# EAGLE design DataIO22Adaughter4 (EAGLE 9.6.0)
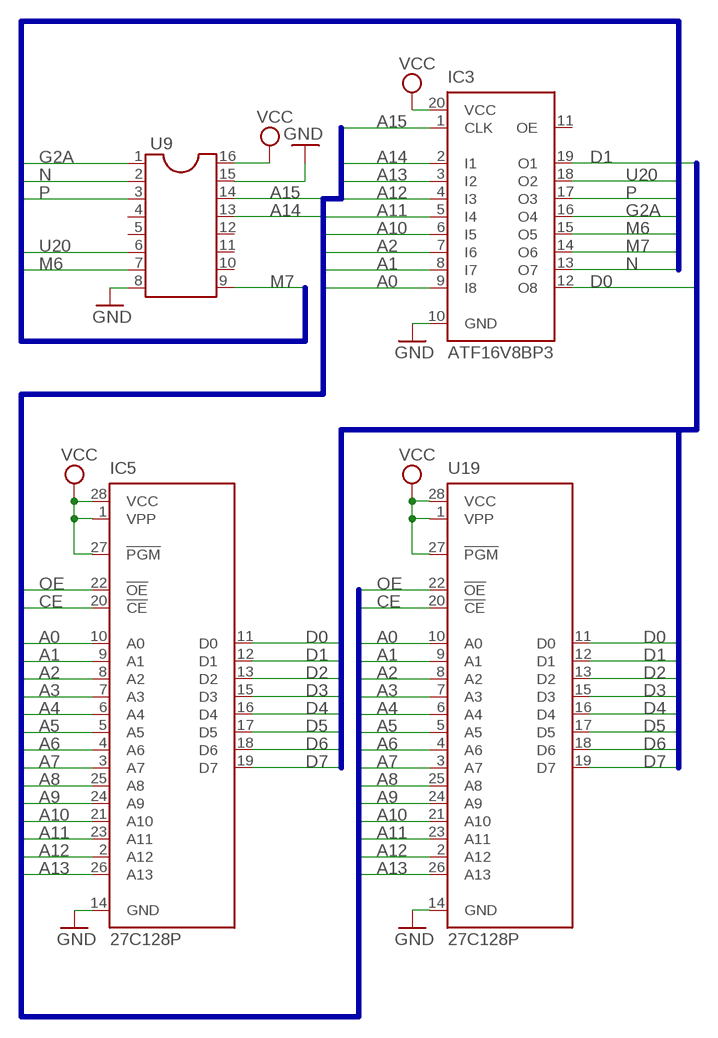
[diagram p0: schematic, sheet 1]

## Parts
IC3  ATF16V8BP3  [DIL20]
IC5  27C128P  [DIL28-6]
U9  DIL16S  [SOCKET-16]
U19  27C128P  [DIL28-6]

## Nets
A0: IC3.9(I8) IC5.10(A0) U19.10(A0)
A1: IC3.8(I7) IC5.9(A1) U19.9(A1)
A2: IC3.7(I6) IC5.8(A2) U19.8(A2)
A3: IC5.7(A3) U19.7(A3)
A4: IC5.6(A4) U19.6(A4)
A5: IC5.5(A5) U19.5(A5)
A6: IC5.4(A6) U19.4(A6)
A7: IC5.3(A7) U19.3(A7)
A8: IC5.25(A8) U19.25(A8)
A9: IC5.24(A9) U19.24(A9)
A10: IC3.6(I5) IC5.21(A10) U19.21(A10)
A11: IC3.5(I4) IC5.23(A11) U19.23(A11)
A12: IC3.4(I3) IC5.2(A12) U19.2(A12)
A13: IC3.3(I2) IC5.26(A13) U19.26(A13)
A14: IC3.2(I1) U9.13
A15: IC3.1(CLK) U9.14
CE: IC5.20(!CE) U19.20(!CE)
D0: IC3.12(O8) IC5.11(D0) U19.11(D0)
D1: IC3.19(O1) IC5.12(D1) U19.12(D1)
D2: IC5.13(D2) U19.13(D2)
D3: IC5.15(D3) U19.15(D3)
D4: IC5.16(D4) U19.16(D4)
D5: IC5.17(D5) U19.17(D5)
D6: IC5.18(D6) U19.18(D6)
D7: IC5.19(D7) U19.19(D7)
G2A: IC3.16(O4) U9.1
GND: IC3.10(GND) IC5.14(GND) U9.8 U9.15 U19.14(GND)
M6: IC3.15(O5) U9.7
M7: IC3.14(O6) U9.9
N: IC3.13(O7) U9.2
OE: IC5.22(!OE) U19.22(!OE)
P: IC3.17(O3) U9.3
U20: IC3.18(O2) U9.6
VCC: IC3.20(VCC) IC5.1(VPP) IC5.27(!PGM) IC5.28(VCC) U9.16 U19.1(VPP) U19.27(!PGM) U19.28(VCC)
Unconnected: IC3.11(OE) U9.4 U9.5 U9.10 U9.11 U9.12

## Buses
A[0..15],CE,OE,PGM
D[0..7]
G2A,M6,M7,N,P,U20

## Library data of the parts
IC3 = atmel:ATF16V8B: High perfomance CMOS (electrically erasable) programmable logic device (PLD) ABLE-Atmel-ABEL - P18V8R, P16V8C, P16V8AS, P17V8 COPL Atmel-WinCUPL - G16V8MS, G16V8MA, G16V8AS, G16V8 LOG/IC - GAL16V8_R, GAL16V8_G7, GAL16V8_C), GAL16V8 Tango-PLD - G16V8R, G16V8C, G16V8AS, G16V8 Source: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; MPN: ATF16V8CZ-15PU; OC_FARNELL: 1551768; OC_NEWARK: 94M6254
IC5 U19 = microchip:27*128: CMOS EPROM 128 K (16 K x 8); OC_FARNELL: unknown; OC_NEWARK: unknown
U9 = ic-package:DIL16: Dual In Line / Socket

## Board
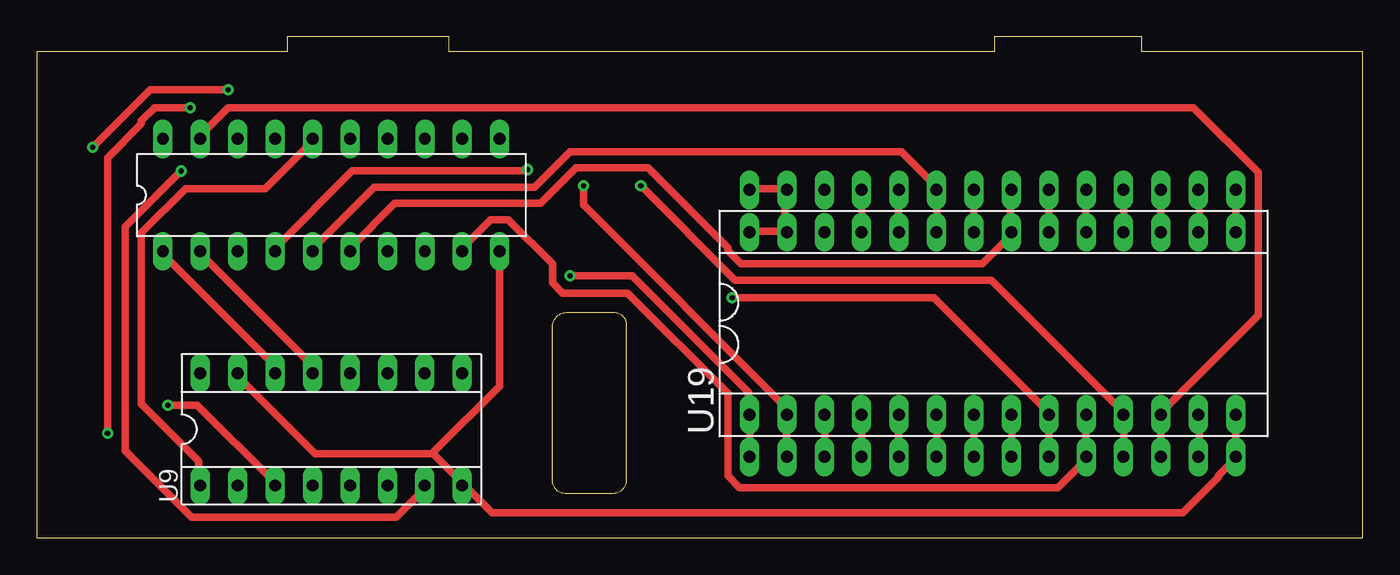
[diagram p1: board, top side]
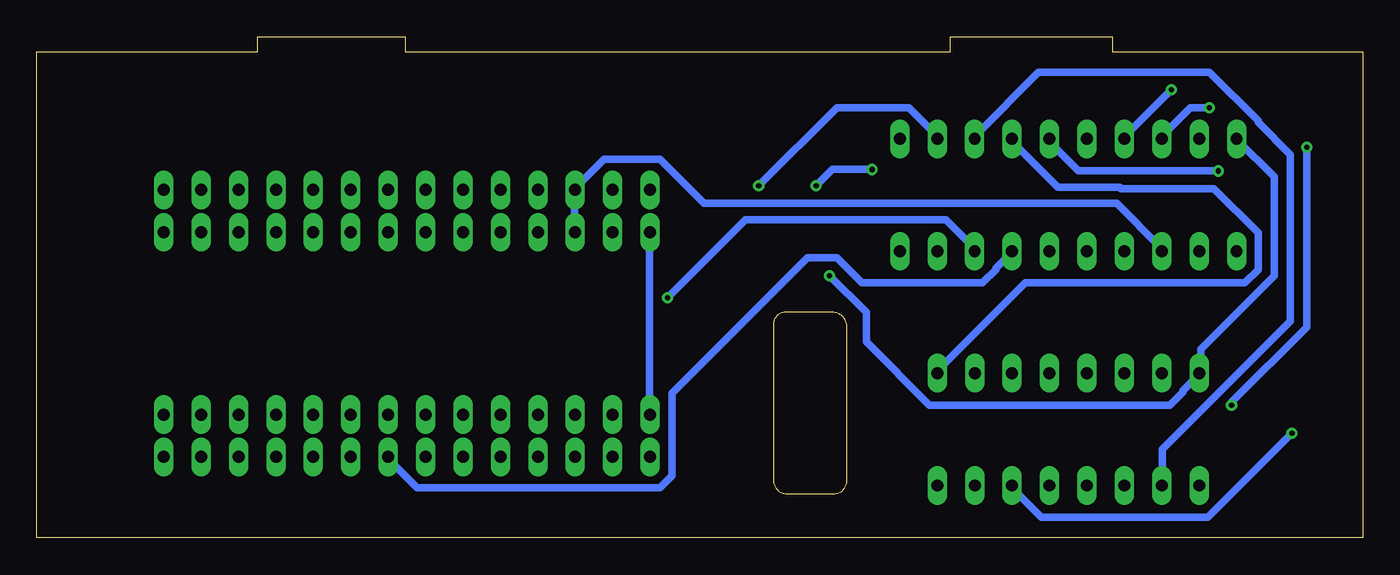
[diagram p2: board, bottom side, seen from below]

Size 90 x 34 mm. Coordinates in mm from the lower left corner, seen from the top.
Outline: 0,0 90,0 90,33 75,33 75,34 65,34 65,33 28,33 28,34 17,34 17,33 0,33 0,0
Copper layers (1*16): Top 0.035mm / dielectric 1.5mm / Bottom 0.035mm
Design rules "default *": minimum track width 20mil, minimum drill 0.35mm, track to track 20mil, track to pad 20mil, pad to pad 20mil, via to via 20mil, smd to smd 20mil, copper to edge 40mil, drill to drill 20mil, minimum pad ring 10mil, minimum via ring 8mil, stop-mask expansion 4mil, vias tented up to drill 0mil, thermal gap 10mil

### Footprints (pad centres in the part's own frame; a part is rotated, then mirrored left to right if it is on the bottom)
DIL20 = drill 0.813 long: 1 -11.43,-3.81; 2 -8.89,-3.81; 3 -6.35,-3.81; 4 -3.81,-3.81; 5 -1.27,-3.81; 6 1.27,-3.81; 7 3.81,-3.81; 8 6.35,-3.81; 9 8.89,-3.81; 10 11.43,-3.81; 11 11.43,3.81; 12 8.89,3.81; 13 6.35,3.81; 14 3.81,3.81; 15 1.27,3.81; 16 -1.27,3.81; 17 -3.81,3.81; 18 -6.35,3.81; 19 -8.89,3.81; 20 -11.43,3.81
DIL28-6 = drill 0.813 long: 1 -16.51,-7.62; 2 -13.97,-7.62; 3 -11.43,-7.62; 4 -8.89,-7.62; 5 -6.35,-7.62; 6 -3.81,-7.62; 7 -1.27,-7.62; 8 1.27,-7.62; 9 3.81,-7.62; 10 6.35,-7.62; 11 8.89,-7.62; 12 11.43,-7.62; 13 13.97,-7.62; 14 16.51,-7.62; 15 16.51,7.62; 16 13.97,7.62; 17 11.43,7.62; 18 8.89,7.62; 19 6.35,7.62; 20 3.81,7.62; 21 1.27,7.62; 22 -1.27,7.62; 23 -3.81,7.62; 24 -6.35,7.62; 25 -8.89,7.62; 26 -11.43,7.62; 27 -13.97,7.62; 28 -16.51,7.62
SOCKET-16 = drill 0.813 long: 1 -8.89,-3.81; 2 -6.35,-3.81; 3 -3.81,-3.81; 4 -1.27,-3.81; 5 1.27,-3.81; 6 3.81,-3.81; 7 6.35,-3.81; 8 8.89,-3.81; 9 8.89,3.81; 10 6.35,3.81; 11 3.81,3.81; 12 1.27,3.81; 13 -1.27,3.81; 14 -3.81,3.81; 15 -6.35,3.81; 16 -8.89,3.81

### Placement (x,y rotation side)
IC3  19.99,23.26 0 top
IC5  64.88,15.99 0 top
U9  19.99,7.37 0 top
U19  64.88,13.12 0 top

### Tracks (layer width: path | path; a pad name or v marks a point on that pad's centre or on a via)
A0
  Top 0.508: IC5.10 71.2,8.3 71.2,5.5 U19.10 71.2,5.3 69.3,3.4 47.7,3.4 46.9,4.2 46.9,9.8 40.1,16.6 35.7,16.6 35,17.3 35,18.6 32,21.6 30.8,21.6 28.9,19.7 28.9,19.5 IC3.9
A1  (via drill 0.35)
  Top 0.508: v47.2,16.3 60.9,16.3 68.6,8.6 68.6,8.4 IC5.9 68.7,8.1 U19.9
  Bottom 0.508: v47.2,16.3 41.9,21.6 28.3,21.6 26.4,19.7 26.4,19.5 IC3.8
A2
  Top 0.508: U19.8 66.2,5.5 66.2,8.3 IC5.8
  Bottom 0.508: IC3.7 23.8,19.4 24.9,18.3 24.9,18.2 25.8,17.3 34,17.3 35.7,19 37.7,19 46.9,9.8 46.9,4.2 47.7,3.4 64.2,3.4 66.1,5.3 66.1,5.5 U19.8
A3
  Top 0.508: U19.7 63.6,8.3 IC5.7
A4
  Top 0.508: U19.6 61.1,5.5 61.1,8.3 IC5.6
A5
  Top 0.508: U19.5 58.5,5.5 58.5,8.3 IC5.5
A6
  Top 0.508: U19.4 56,8.3 IC5.4
A7
  Top 0.508: U19.3 53.5,5.5 53.5,8.3 IC5.3
A8
  Top 0.508: U19.25 56,20.8 IC5.25
A9
  Top 0.508: U19.24 58.5,20.8 58.5,23.6 IC5.24
A10
  Top 0.508: IC3.6 21.3,19.5 21.3,19.7 24.3,22.7 34.2,22.7 36.6,25.1 41.5,25.1 46.9,19.7 46.9,19.5 47.8,18.6 64.2,18.6 66.1,20.5 66.1,20.7 U19.21 66.1,21 66.1,23.6 IC5.21
A11
  Top 0.508: IC3.5 18.8,19.5 18.8,19.7 22.9,23.8 33.8,23.8 36.2,26.2 58.7,26.2 61,23.9 61,23.7 IC5.23 61.1,23.4 61.1,20.8 U19.23
A12  (via drill 0.35)
  Top 0.508: U19.2 50.9,8.3 IC5.2 50.8,8.6 50.8,8.9 37.1,22.6 v37.1,23.9 | v33.3,25 33.2,24.9 21.4,24.9 16.2,19.7 16.2,19.5 IC3.4
  Bottom 0.508: v33.3,25 36,25 v37.1,23.9
A13
  Bottom 0.508: IC3.3 13.7,19.5 13.7,19.7 16.7,22.7 44.7,22.7 47.7,25.7 51.5,25.7 53.5,23.7 IC5.26 53.5,23.4 53.5,20.8 U19.26
A14
  Top 0.508: U9.13 18.7,11.2 18.7,11.7 11.1,19.3 11.1,19.4 IC3.2
A15
  Top 0.508: U9.14 16.1,11.2 16.1,11.7 8.6,19.2 8.6,19.4 IC3.1
CE
  Top 0.508: U19.20 68.7,20.8 IC5.20
D0  (via drill 0.35)
  Top 0.508: U19.11 73.8,5.5 73.8,8.3 IC5.11 73.7,8.6 64.8,17.5 47.4,17.5 v41,23.9
  Bottom 0.508: v41,23.9 35.7,29.2 30.8,29.2 28.9,27.3 28.9,27.1 IC3.12
D1
  Top 0.508: U19.12 76.3,8.3 IC5.12 76.4,8.6 82.9,15.1 82.9,24.8 78.5,29.2 13,29.2 11.1,27.3 11.1,27.1 IC3.19
D2
  Top 0.508: U19.13 78.9,5.5 78.9,8.3 IC5.13
D3
  Top 0.508: U19.15 81.4,20.8 IC5.15
D4
  Top 0.508: U19.16 78.9,20.8 78.9,23.6 IC5.16
D5
  Top 0.508: U19.17 76.3,20.8 IC5.17
D6
  Top 0.508: U19.18 73.8,20.8 73.8,23.6 IC5.18
D7
  Top 0.508: U19.19 71.2,20.8 71.2,23.6 IC5.19
G2A
  Top 0.508: U9.1 11,3.6 11,5.2 7.1,9.1 7.1,20.7 10.1,23.7 15.5,23.7 18.8,27 IC3.16
GND
  Top 0.508: IC5.14 81.4,8.3 U19.14 81.3,5.3 80.2,4.2 80.2,4.1 77.8,1.7 30.9,1.7 29.1,3.5 U9.8 28.8,3.6 28.8,3.8 26.9,5.7 | 26.9,5.7 18.9,5.7 13.7,10.9 13.7,11.1 U9.15 | IC3.10 31.4,19.4 31.4,10.3 27,5.9 26.9,5.7
M6  (via drill 0.35)
  Top 0.508: v9.8,24.9 6,21.1 6,5.9 10.5,1.4 24.4,1.4 26.3,3.3 26.3,3.5 U9.7
  Bottom 0.508: v9.8,24.9 19.3,24.9 21.2,26.8 21.2,27 IC3.15
M7
  Bottom 0.508: U9.9 28.8,11.2 28.8,11.4 22.9,17.3 8,17.3 7.1,18.2 7.1,20.7 10.1,23.7 16.4,23.7 16.5,23.8 20.7,23.8 23.8,26.9 23.8,27 IC3.14
N
  Bottom 0.508: U9.2 13.6,3.6 13.6,6 4.9,14.7 4.9,26 7.1,28.2 7.1,28.3 10.4,31.6 22,31.6 26.3,27.3 26.3,27.1 IC3.13
OE
  Top 0.508: U19.22 63.6,20.8 IC5.22
P  (via drill 0.35)
  Top 0.508: v8.9,9 10.9,9 16.1,3.8 16.1,3.6 U9.3 | v3.8,26.5 7.7,30.4 v13,30.4
  Bottom 0.508: v8.9,9 8.9,9.2 3.8,14.3 v3.8,26.5 | v13,30.4 16.1,27.3 16.1,27.1 IC3.17
U20  (via drill 0.35)
  Top 0.508: v4.8,7.1 4.8,25.8 7.1,28.1 7.1,28.3 8,29.2 v10.4,29.2
  Bottom 0.508: v4.8,7.1 10.5,1.4 21.8,1.4 23.7,3.3 23.7,3.5 U9.6 | v10.4,29.2 11.7,29.2 13.6,27.3 13.6,27.1 IC3.18
VCC  (via drill 0.35)
  Top 0.508: U19.1 48.4,5.5 48.4,8.3 IC5.1 48.3,8.6 48.3,9.9 40.4,17.8 v36.2,17.8 | U19.28 48.4,20.8 50.9,20.8 U19.27 50.8,21 50.8,23.4 IC5.27 50.9,23.7 48.4,23.7 IC5.28
  Bottom 0.508: IC3.20 8.5,27 6,24.5 6,17.8 11,12.8 11,11.2 U9.16 11.2,11 12.2,10 12.2,9.9 13.1,9 29.4,9 33.7,13.3 33.7,15.3 v36.2,17.8 | IC5.1 48.4,8.4 48.4,20.7 U19.28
